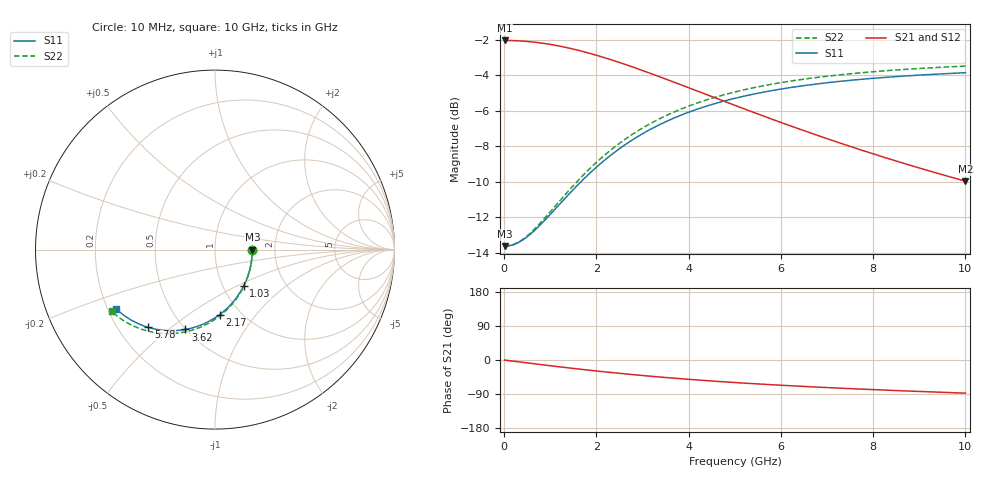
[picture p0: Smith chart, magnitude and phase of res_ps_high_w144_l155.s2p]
! Created Wed Nov  4 11:48:21 2020
# ghz S ma R 50
! 2 Port Network Data from SP1.SP block
! freq  magS11  angS11  magS21  angS21  magS12  angS12  magS22  angS22
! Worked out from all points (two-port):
!   1000 points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, 10 MHz to 10 GHz, reference 50 ohm
!   highest |S21| = -2.03 dB at 10 MHz (marker M1); lowest = -10.0 dB at 10 GHz (marker M2)
!   |S21| within 3 dB of the highest: start of sweep to 4.334 GHz
!   lowest |S11| = -13.6 dB at 10 MHz (marker M3), VSWR 1.53, Z = 76.3 - j0.143 ohm
!   |S11| at or under -10 dB: start of sweep to 1.665 GHz
!   |S22| runs from -13.6 to -3.5 dB; largest |S21 - S12| = 0
!   S11 on the Smith chart (normalised r, x): 10 MHz: 1.53, -0.00; 1.03 GHz: 1.25, -0.54; 2.17 GHz: 0.80, -0.67; 3.62 GHz: 0.50, -0.57; 5.78 GHz: 0.33, -0.42; 10 GHz: 0.23, -0.26
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0.01  0.2081 -0.2  0.7919 -0.2  0.7919 -0.2  0.2081 -0.3
0.06  0.2082 -3.1  0.7919 -1.0  0.7919 -1.0  0.2082 -3.3
0.22  0.2106 -12.3  0.791 -3.4  0.791 -3.4  0.2108 -12.7
0.44  0.2183 -24.4  0.788 -6.8  0.788 -6.8  0.2193 -25.2
0.69  0.2324 -37.0  0.7822 -10.6  0.7822 -10.6  0.2348 -38.0
1.03  0.2583 -51.9  0.7707 -15.6  0.7707 -15.6  0.2628 -53.1
1.36  0.2876 -63.9  0.7558 -20.3  0.7558 -20.3  0.2945 -65.1
1.68  0.3177 -73.7  0.7387 -24.7  0.7387 -24.7  0.3267 -74.8
2.17  0.3632 -85.9  0.7084 -31.2  0.7084 -31.2  0.3752 -87.0
2.45  0.3878 -91.8  0.6897 -34.6  0.6897 -34.6  0.4014 -92.7
2.73  0.4111 -97.0  0.6704 -37.9  0.6704 -37.9  0.4261 -97.9
3.03  0.4343 -102.0  0.6494 -41.3  0.6494 -41.3  0.4507 -102.8
3.34  0.4563 -106.6  0.6277 -44.6  0.6277 -44.6  0.4741 -107.3
3.62  0.4745 -110.4  0.6083 -47.4  0.6083 -47.4  0.4934 -111.0
4.26  0.5106 -117.8  0.5654 -53.4  0.5654 -53.4  0.5315 -118.3
5.01  0.5442 -124.8  0.519 -59.5  0.519 -59.5  0.567 -125.2
5.78  0.571 -130.6  0.4762 -65.1  0.4762 -65.1  0.5953 -131.0
6.67  0.5945 -136.1  0.4329 -70.8  0.4329 -70.8  0.6201 -136.3
7.47  0.6106 -140.1  0.3991 -75.4  0.3991 -75.4  0.6372 -140.3
8.34  0.6242 -143.7  0.3672 -79.9  0.3672 -79.9  0.6515 -143.9
9.16  0.6341 -146.6  0.341 -83.8  0.341 -83.8  0.662 -146.7
10  0.6421 -149.1  0.3175 -87.5  0.3175 -87.5  0.6705 -149.1
